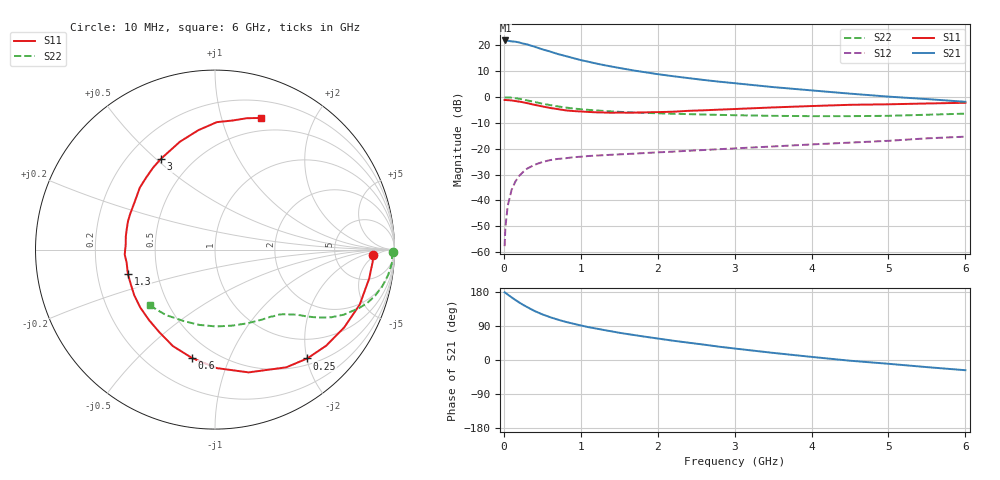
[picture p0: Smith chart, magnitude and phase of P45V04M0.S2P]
! SIEMENS Small Signal Semiconductors
! BFP182
! Si NPN RF Bipolar Junction Transistor in SOT143
! VCE = 5 V  IC = 4 mA
! Common Emitter S-Parameters:  March  1996
# GHz  S  MA  R  50
!  f  S11  S21  S12  S22
! GHz  MAG  ANG  MAG  ANG  MAG  ANG  MAG  ANG
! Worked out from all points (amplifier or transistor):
!   36 points, 10 MHz to 6 GHz, reference 50 ohm
!   highest |S21| = 21.9 dB at 20 MHz (marker M1)
!   |S21| within 3 dB of that: start of sweep to 456.7 MHz
!   unconditionally stable (mu >= 1): 1.779 GHz to 5.718 GHz
!   at 250 MHz: K = 0.18, MSG = 24.9 dB, |S12| = -29.0 dB
!   at 1.4 GHz: K = 0.85, MSG = 17.1 dB, |S12| = -22.3 dB
!   at 6 GHz: K = 0.96, MSG = 6.8 dB, |S12| = -15.3 dB
!   S11 on the Smith chart (normalised r, x): 10 MHz: 14, -4; 250 MHz: 0.61, -2.01; 600 MHz: 0.38, -0.74; 1.3 GHz: 0.34, -0.12; 3 GHz: 0.34, +0.52; 6 GHz: 0.36, +1.35
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0.01  0.8797 -2.1  12.28 178.5  0.0013 86.7  0.9925 -0.8
0.02  0.8812 -4.4  12.51 177.4  0.003 87.9  0.9864 -1.7
0.05  0.874 -10.6  12.34 172.7  0.0078 87.7  0.9888 -4.3
0.15  0.8402 -31.1  11.84 158.4  0.0232 72.1  0.9541 -12.4
0.2  0.8189 -40.8  11.43 151.8  0.0299 68.6  0.9283 -16.1
0.25  0.795 -49.7  10.9 145.6  0.0355 63.9  0.899 -19.3
0.3  0.7668 -58.8  10.52 140.0  0.041 59.4  0.8664 -22.1
0.4  0.7092 -74.7  9.464 129.2  0.049 52.4  0.804 -26.8
0.5  0.6603 -89.2  8.422 120.5  0.0553 47.1  0.7496 -30.2
0.6  0.6175 -101.9  7.639 113.1  0.0603 42.7  0.7012 -32.7
0.7  0.5867 -113.5  6.849 106.6  0.0636 39.4  0.6622 -34.6
0.8  0.5554 -123.8  6.26 100.8  0.0655 36.9  0.6298 -36.2
1  0.5269 -142.1  5.214 91.2  0.0702 33.4  0.5834 -38.5
1.1  0.517 -150.4  4.842 86.7  0.0724 32.3  0.5665 -39.7
1.3  0.5042 -164.3  4.172 79.2  0.0751 30.1  0.5399 -41.8
1.6  0.4983 177.0  3.461 68.7  0.0792 29.4  0.5105 -45.1
2.2  0.5219 148.5  2.543 50.9  0.088 28.5  0.4773 -53.2
3  0.5884 120.9  1.861 30.3  0.1017 27.7  0.4468 -67.2
3.5  0.6317 108.1  1.564 18.8  0.1109 26.4  0.434 -77.5
4.5  0.7101 89.2  1.168 -1.9  0.1316 23.1  0.4284 -101.5
5.5  0.7531 76.4  0.916 -18.8  0.1592 18.9  0.456 -127.0
6  0.7772 70.7  0.813 -27.0  0.1716 15.0  0.4788 -139.6
